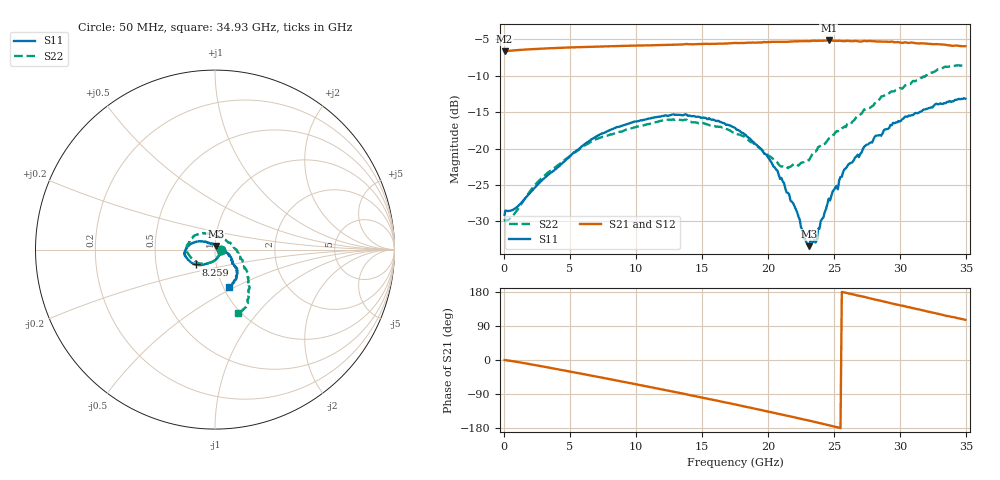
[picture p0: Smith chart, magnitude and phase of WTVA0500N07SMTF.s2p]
! 50 ohm 2-Port S-parameters measured by Modelithics Inc support@modelithics.com  Tampa, FL USA 813-866-6335 (February 2024)
! Smiths Interconnect,  5dB P/N: WTVA0500N07SMTF, Temperature: 0 C
! Board: 10 mil Rogers 4350B, Mounting Pad Dimensions: Length: 15 mils, Width: 25 mils, Gap: 40 mils.
# Hz S RI R 50
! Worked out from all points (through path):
!   352 points, 50 MHz to 34.93 GHz, reference 50 ohm
!   highest |S21| = -5.15 dB at 24.58 GHz (marker M1); lowest = -6.6 dB at 50 MHz (marker M2)
!   group delay of S21, straight-line fit = 20.5 ps
!   lowest |S11| = -33.4 dB at 23.09 GHz (marker M3), VSWR 1.04, Z = 50.4 + j2.11 ohm
!   |S11| at or under -10 dB: start of sweep to end of sweep
!   |S22| runs from -30.0 to -8.5 dB; largest |S21 - S12| = 0.0034
!   S11 on the Smith chart (normalised r, x): 50 MHz: 1.07, -0.00; 8.259 GHz: 0.79, -0.13; 34.93 GHz: 1.06, -0.46
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5e7  0.035 -0.00164  0.4661 -0.00131  0.4658 -0.00144  0.0329 -0.00125
6.975e8  0.03 -0.0234  0.4709 -0.0274  0.4707 -0.0274  0.0249 -0.0243
2.787e9  0.0001 -0.0595  0.466 -0.1346  0.4657 -0.1346  -0.00395 -0.0618
5.8715e9  -0.0613 -0.083  0.4012 -0.2941  0.4009 -0.2941  -0.0643 -0.0784
8.2595e9  -0.1086 -0.0828  0.3088 -0.3991  0.3081 -0.3992  -0.107 -0.0663
1.1742e10  -0.1596 -0.0444  0.1226 -0.4987  0.1218 -0.4986  -0.1529 -0.0176
1.3732e10  -0.1707 -0.0196  0.000299 -0.521  -5.16e-05 -0.5207  -0.1565 0.0215
1.7513e10  -0.1342 0.0331  -0.2454 -0.4708  -0.2457 -0.4704  -0.0954 0.0863
2.0697e10  -0.055 0.0445  -0.424 -0.3364  -0.4242 -0.3355  0.000148 0.0802
2.1493e10  -0.0335 0.0366  -0.4564 -0.2912  -0.4564 -0.2906  0.0251 0.0689
2.2687e10  -0.0012 0.0242  -0.502 -0.2139  -0.5018 -0.2133  0.0653 0.0473
2.3085e10  0.00408 0.021  -0.513 -0.1868  -0.5127 -0.1866  0.0739 0.0381
2.33835e10  0.0126 0.0189  -0.5236 -0.1679  -0.5234 -0.1675  0.0846 0.039
2.3682e10  0.0187 0.0143  -0.5292 -0.1441  -0.5288 -0.144  0.0931 0.029
2.37815e10  0.0247 0.0136  -0.5328 -0.1375  -0.5326 -0.1371  0.0991 0.0259
2.45775e10  0.0453 -0.00221  -0.5474 -0.0759  -0.5471 -0.0754  0.1169 0.00197
2.5274e10  0.0512 -0.0119  -0.5486 -0.0213  -0.5483 -0.0212  0.1296 -0.0222
2.5473e10  0.0614 -0.0172  -0.5495 -0.00397  -0.5492 -0.00407  0.1309 -0.0264
2.607e10  0.0737 -0.0248  -0.5477 0.0405  -0.5473 0.0408  0.1418 -0.0453
2.91545e10  0.1073 -0.0873  -0.4728 0.2627  -0.472 0.2632  0.1826 -0.156
3.27365e10  0.1153 -0.1675  -0.2833 0.438  -0.2835 0.4374  0.1829 -0.2915
3.49255e10  0.0762 -0.2062  -0.1397 0.4849  -0.1374 0.4851  0.1275 -0.3534
